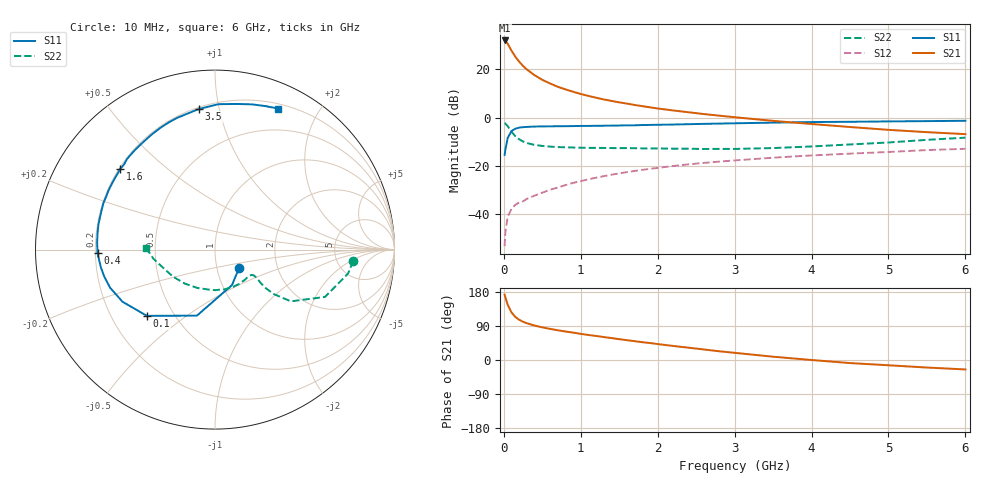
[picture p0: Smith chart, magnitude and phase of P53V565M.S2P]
! SIEMENS Small Signal Semiconductors
! BFP183
! Si NPN RF Bipolar Junction Transistor in SOT143
! VCE = 3.5 V  IC = 65 mA
! Common Emitter S-Parameters:  March  1996
# GHz  S  MA  R  50
!  f  S11  S21  S12  S22
! GHz  MAG  ANG  MAG  ANG  MAG  ANG  MAG  ANG
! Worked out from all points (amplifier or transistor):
!   36 points, 10 MHz to 6 GHz, reference 50 ohm
!   highest |S21| = 31.9 dB at 10 MHz (marker M1)
!   |S21| within 3 dB of that: start of sweep to 78.32 MHz
!   unconditionally stable (mu >= 1): start of sweep to 28.59 MHz; 208.7 MHz to end of sweep
!   at 250 MHz: K = 1.14, MAG = 25.7 dB, |S12| = -34.6 dB
!   at 1.4 GHz: K = 1.64, MAG = 10.6 dB, |S12| = -23.6 dB
!   at 6 GHz: K = 1.22, MAG = 0.2 dB, |S12| = -12.9 dB
!   S11 on the Smith chart (normalised r, x): 10 MHz: 1.28, -0.27; 100 MHz: 0.35, -0.36; 400 MHz: 0.21, -0.02; 1.6 GHz: 0.20, +0.36; 3.5 GHz: 0.21, +0.87; 6 GHz: 0.25, +1.51
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0.01  0.1695 -38.0  39.43 172.5  0.0022 65.3  0.7724 -4.7
0.02  0.2193 -64.5  38.62 165.3  0.0043 69.5  0.7534 -10.2
0.05  0.3815 -105.3  33.62 145.8  0.0089 61.3  0.667 -23.3
0.1  0.5294 -135.8  24.21 125.3  0.013 49.6  0.5115 -34.3
0.15  0.5917 -150.6  18.14 113.5  0.0158 48.4  0.4117 -37.1
0.2  0.6221 -160.1  14.29 106.1  0.0176 48.9  0.3553 -37.2
0.25  0.6352 -166.4  11.69 100.8  0.0186 50.1  0.3214 -36.4
0.3  0.6436 -171.2  9.882 97.0  0.021 51.1  0.2978 -35.2
0.4  0.6547 -178.2  7.528 90.8  0.0244 55.5  0.273 -33.9
0.5  0.6579 176.6  6.044 86.2  0.0281 56.6  0.2596 -33.7
0.6  0.6608 171.9  5.092 82.1  0.0322 59.1  0.2517 -34.2
0.7  0.6641 167.8  4.347 78.5  0.0359 60.4  0.2462 -35.0
0.9  0.6687 160.9  3.431 72.3  0.0447 61.9  0.2413 -38.0
1.1  0.6742 154.0  2.814 66.0  0.0532 61.8  0.2371 -41.7
1.3  0.6807 148.3  2.376 60.5  0.0617 61.0  0.2363 -46.3
1.6  0.6938 139.5  1.949 52.3  0.0748 59.6  0.2345 -53.3
2.2  0.7198 124.0  1.408 37.1  0.0999 54.3  0.228 -70.3
2.8  0.7538 110.1  1.099 23.0  0.1232 48.3  0.2261 -89.7
3.5  0.7884 96.6  0.857 8.7  0.1485 41.5  0.235 -114.3
4.5  0.8211 81.2  0.64 -8.1  0.1802 31.3  0.2789 -147.5
5.5  0.8473 70.7  0.501 -19.9  0.2136 22.0  0.3472 -171.7
6  0.8609 65.9  0.456 -24.9  0.227 16.8  0.3857 178.3
